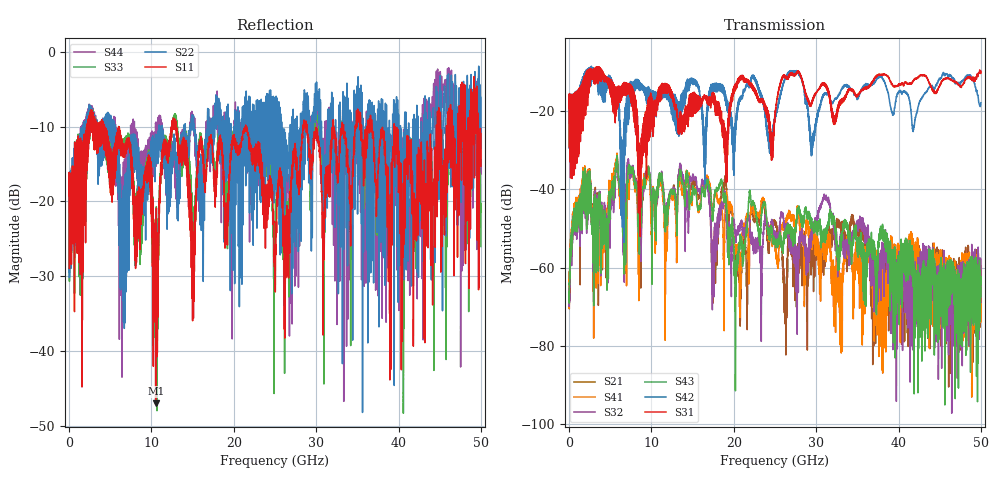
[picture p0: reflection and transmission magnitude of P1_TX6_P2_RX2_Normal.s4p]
!Keysight Technologies,N5225B,MY57041031,A.13.20.10
!Date: Friday, May 31, 2019 11:30:21
!Correction: S11(Full 4 Port(1,2,3,4))
!S12(Full 4 Port(1,2,3,4))
!S13(Full 4 Port(1,2,3,4))
!S14(Full 4 Port(1,2,3,4))
!S21(Full 4 Port(1,2,3,4))
!S22(Full 4 Port(1,2,3,4))
!S23(Full 4 Port(1,2,3,4))
!S24(Full 4 Port(1,2,3,4))
!S31(Full 4 Port(1,2,3,4))
!S32(Full 4 Port(1,2,3,4))
!S33(Full 4 Port(1,2,3,4))
!S34(Full 4 Port(1,2,3,4))
!S41(Full 4 Port(1,2,3,4))
!S42(Full 4 Port(1,2,3,4))
!S43(Full 4 Port(1,2,3,4))
!S44(Full 4 Port(1,2,3,4))
!S4P File: Measurements: <S11,S12,S13,S14>,
!<S21,S22,S23,S24>,
!<S31,S32,S33,S34>,
!<S41,S42,S43,S44>:
# Hz S  dB  R 50.0
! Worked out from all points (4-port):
!   5000 points, 10 MHz to 50 GHz, reference 50 ohm
!   strongest paths, dB at 10 MHz, 12.51 GHz, 25.01 GHz, 37.51 GHz, 50 GHz:
!     S31: -19.3, -15.4, -21.6, -10.8, -9.9
!     S42: -19.4, -15.9, -21.6, -11.2, -17.9
!     S43: -66.1, -40.9, -53.6, -55.2, -63.5
!     S32: -65.3, -40.7, -50.7, -57.3, -68.9
!     S41: -61.6, -42.3, -54.6, -64.3, -59.4
!     S21: -66.7, -40.9, -48.2, -61.4, -65.6
!   lowest |S11| = -47.0 dB at 10.52 GHz (marker M1), VSWR 1.01, Z = 49.6 - j0.0452 ohm
!   |S11| at or under -10 dB: 6.02 GHz to 12.47 GHz (6.445 GHz wide, 69.7 % of centre); 13.02 GHz to 21.43 GHz (8.402 GHz wide, 48.8 % of centre); 21.46 GHz to 28.42 GHz (6.959 GHz wide, 27.9 % of centre)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
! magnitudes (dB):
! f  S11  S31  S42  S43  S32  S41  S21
! 10 MHz  -19.2  -19.3  -19.4  -66.1  -65.3  -61.6  -66.7
! 1.82 GHz  -16.6  -17.5  -14.9  -37.7  -38.0  -36.8  -37.7
! 6.46 GHz  -12.2  -14.3  -28.9  -43.6  -41.7  -41.9  -42.3
! 10.52 GHz  -47.0  -18.4  -15.2  -48.1  -47.6  -49.1  -47.8
! 12.81 GHz  -9.1  -17.9  -16.7  -41.1  -40.0  -42.2  -39.9
! 26.23 GHz  -25.8  -11.1  -11.8  -51.3  -50.4  -48.9  -69.8
! 50 GHz  -10.9  -9.9  -17.9  -63.5  -68.9  -59.4  -65.6
